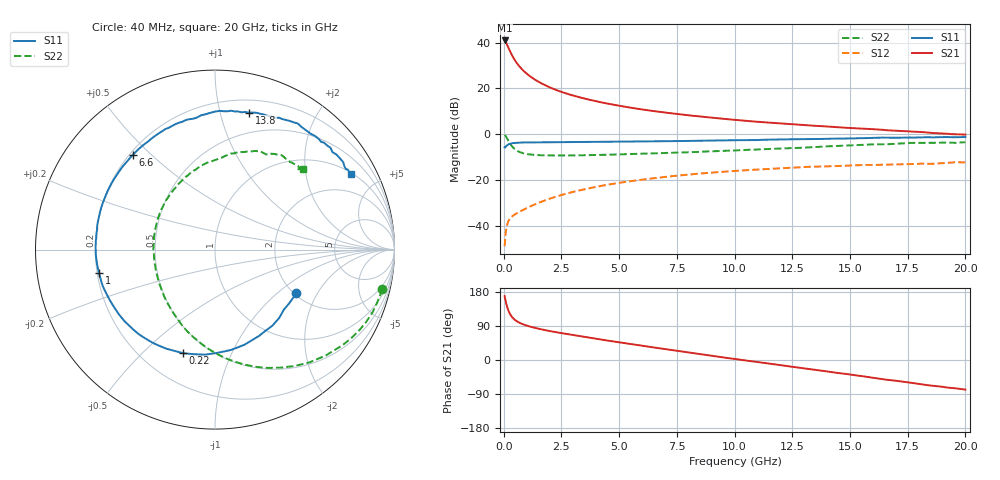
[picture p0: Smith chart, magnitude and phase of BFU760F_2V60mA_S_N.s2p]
! Filename:  P:\Prog\Test\Noise\ATS_data\Testdata_Net\BFU760\BFU760F_2W_C1_2V60mA_D.s2p
! Date/Time: Mon 06/Feb/2012 15:05:47
! BFU760_2W_C1_2V60mA
! bias mode 1: Vout= 1.9999 V, Iout=60.0800 mA, Vin= 0.7996 V, Iin= 0.2261 mA
! Date/time Fri Mar 18 15:18:19 2011
! Device data file deembeded for feedlines and parallel
! Original file: \BFU760\BFU760_2W_C1_2V60mA_R.s2p
! Feed-files: PR003V01_101208_Feed1.s2p, PR003V01_101208_Feed2.s2p
! Parallel-file: PR003V01_101208_Par.s2p
# MHz S MA R 50
!  Freq-MHz  S11-mag  S11-arg  S21-mag  S21-arg  S12-mag  S12-arg  S22-mag  S22-arg
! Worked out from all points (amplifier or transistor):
!   167 points, 40 MHz to 20 GHz, reference 50 ohm
!   highest |S21| = 40.9 dB at 40 MHz (marker M1)
!   |S21| within 3 dB of that: start of sweep to 197.5 MHz
!   unconditionally stable (mu >= 1): 2.826 GHz to 14.03 GHz; 14.31 GHz to 14.86 GHz
!   at 550 MHz: K = 0.53, MSG = 33.0 dB, |S12| = -34.7 dB
!   at 4.2 GHz: K = 1.03, MAG = 17.2 dB, |S12| = -22.6 dB
!   at 20 GHz: K = 0.94, MSG = 6.1 dB, |S12| = -12.3 dB
!   lowest NFmin = 0.82 dB at 1.2 GHz
!   S11 on the Smith chart (normalised r, x): 40 MHz: 2.06, -1.36; 220 MHz: 0.37, -0.67; 1 GHz: 0.21, -0.10; 6.6 GHz: 0.21, +0.44; 13.8 GHz: 0.31, +1.23; 20 GHz: 1.05, +3.56
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40  0.5147 -28.1  111.5 168.6  0.00357 80.4  0.9585 -13.4
50  0.5103 -36.1  110.2 164.8  0.003942 77.9  0.9507 -18.0
80  0.5308 -52.8  105.4 156.5  0.006508 72.1  0.9196 -29.6
120  0.5552 -72.9  96.64 146.3  0.008958 64.9  0.8541 -43.6
160  0.5759 -88.9  87.11 138.0  0.01093 59.0  0.7857 -55.6
220  0.6037 -107.0  74.56 128.1  0.01302 53.1  0.6926 -70.6
280  0.6196 -120.2  63.89 120.8  0.01447 49.4  0.618 -82.7
340  0.6315 -130.0  55.42 115.2  0.01559 47.2  0.5597 -92.8
400  0.6378 -137.5  48.65 110.8  0.01651 46.1  0.5152 -101.1
480  0.6449 -145.2  41.63 106.2  0.01759 45.6  0.4726 -110.6
700  0.6534 -158.2  29.5 97.9  0.02037 47.0  0.4051 -129.1
1000  0.6595 -168.5  20.93 90.8  0.02429 50.0  0.3686 -145.2
1400  0.6645 -177.2  15.04 84.2  0.02993 52.8  0.351 -158.8
1850  0.6659 175.9  11.38 78.2  0.03671 54.3  0.3437 -169.1
3400  0.6757 159.1  6.179 61.9  0.06104 51.9  0.3465 168.9
6600  0.6992 131.1  3.144 32.3  0.1105 35.3  0.3813 137.9
6800  0.7002 129.5  3.052 30.5  0.1134 34.0  0.3841 136.1
10200  0.7391 102.9  2.017 1.1  0.1593 12.0  0.4464 108.5
13400  0.7789 79.1  1.531 -25.2  0.1948 -10.2  0.5193 84.8
13800  0.7863 76.1  1.494 -28.5  0.1978 -13.1  0.5325 82.1
16800  0.8361 53.6  1.2 -53.4  0.2169 -32.6  0.6082 60.7
20000  0.8665 29.1  0.9788 -78.1  0.2429 -54.4  0.6658 42.5
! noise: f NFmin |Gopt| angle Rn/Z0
400  0.8274  0.4181  181.9  0.0387
700  0.8227  0.422  184.2  0.0397
1100  0.8197  0.4276  187.2  0.0412
1500  0.8202  0.4337  190.1  0.0429
1900  0.8244  0.4402  193  0.0449
2300  0.8321  0.4472  195.8  0.0472
2900  0.8505  0.4585  200  0.0509
3800  0.8932  0.4776  206.1  0.0576
4600  0.9465  0.4966  211.4  0.0646
6000  1.074  0.5351  220.3  0.079
